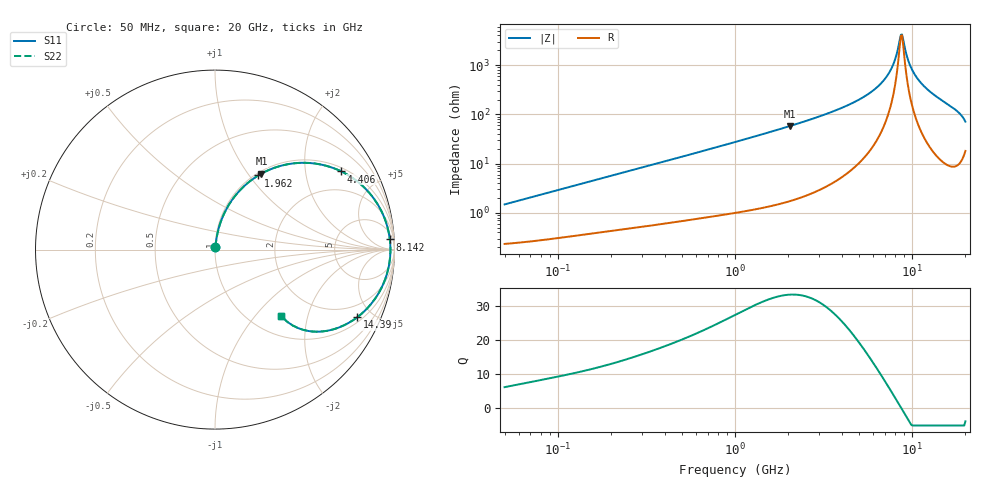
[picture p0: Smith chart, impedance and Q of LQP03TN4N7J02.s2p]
!Murata Part Number: LQP03TN4N7J02
!These Parameters are Measured in Series Mode Connection
!  o--[Z]--o
!Port1  Port2
!  o-------o
!Freq. Start=50[MHz] Stop=20[GHz], 401[Steps]
# Hz S RI R 50
!Freq.(Hz) S11(Real) S11(Imag) S21(Real) S21(Imag) S12(Real) S12(Imag) S22(Real) S22(Imag)
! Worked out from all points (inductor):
!   401 points, 50 MHz to 20 GHz, reference 50 ohm
!   read as one part in series: L = 4.63 nH near 51.52 MHz
!   highest Q = 33.5 at 2.052 GHz (marker M1), where L = 4.51 nH
!   self-resonance near 8.645 GHz
!   S11 on the Smith chart (normalised r, x): 50 MHz: 1.00, +0.03; 1.962 GHz: 1.03, +1.11; 4.406 GHz: 1.14, +3.14; 8.142 GHz: 12, +29; 14.39 GHz: 1.24, -4.07; 20 GHz: 1.36, -1.37
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5e7  0.00254 0.0146  0.9975 -0.0146  0.9975 -0.0146  0.00254 0.0146
1.364002e8  0.00503 0.0384  0.995 -0.0384  0.995 -0.0384  0.00503 0.0384
3.721004e8  0.016 0.1004  0.984 -0.1004  0.984 -0.1004  0.016 0.1004
1e9  0.0774 0.2497  0.9226 -0.2497  0.9226 -0.2497  0.0774 0.2497
1.962148e9  0.2411 0.413  0.7589 -0.413  0.7589 -0.413  0.2411 0.413
2.05233e9  0.2591 0.4234  0.7409 -0.4234  0.7409 -0.4234  0.2591 0.4234
2.728004e9  0.3979 0.4742  0.6021 -0.4742  0.6021 -0.4742  0.3979 0.4742
4.405649e9  0.7042 0.4353  0.2958 -0.4353  0.2958 -0.4353  0.7042 0.4353
6.034176e9  0.8865 0.2821  0.1135 -0.2821  0.1135 -0.2821  0.8865 0.2821
6.802353e9  0.9346 0.1987  0.0654 -0.1987  0.0654 -0.1987  0.9346 0.1987
7.442007e9  0.9596 0.1297  0.0404 -0.1297  0.0404 -0.1297  0.9596 0.1297
7.784049e9  0.9682 0.0936  0.0318 -0.0936  0.0318 -0.0936  0.9682 0.0936
8.141811e9  0.974 0.0568  0.026 -0.0568  0.026 -0.0568  0.974 0.0568
8.516016e9  0.977 0.0194  0.023 -0.0194  0.023 -0.0194  0.977 0.0194
8.774992e9  0.9774 -0.00567  0.0226 0.00567  0.0226 0.00567  0.9774 -0.00567
8.907419e9  0.9771 -0.0182  0.0229 0.0182  0.0229 0.0182  0.9771 -0.0182
9.600142e9  0.9705 -0.081  0.0295 0.081  0.0295 0.081  0.9705 -0.081
1.050288e10  0.9517 -0.1551  0.0483 0.1551  0.0483 0.1551  0.9517 -0.1551
1.201863e10  0.9012 -0.2595  0.0988 0.2595  0.0988 0.2595  0.9012 -0.2595
1.438523e10  0.7924 -0.3771  0.2076 0.3771  0.2076 0.3771  0.7924 -0.3771
1.774144e10  0.5863 -0.4568  0.4137 0.4568  0.4137 0.4568  0.5863 -0.4568
2e10  0.3669 -0.3681  0.6331 0.3681  0.6331 0.3681  0.3669 -0.3681
